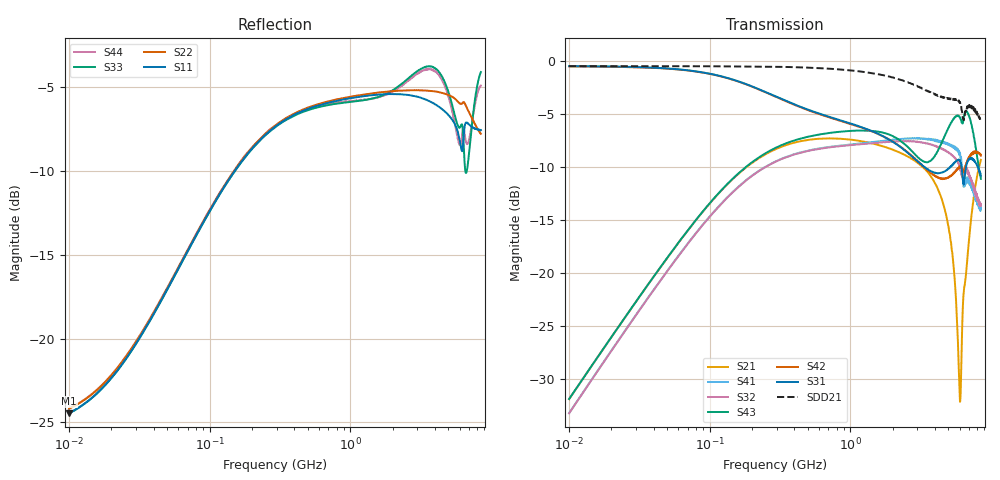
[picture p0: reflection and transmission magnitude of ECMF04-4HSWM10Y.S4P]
!ECMF04-4HSWM10Y
!Typical device
!P1 -OOOOOOO- P3
!P2 -OOOOOOO- P4
!Agilent Technologies,E5071C,MY46109436,A.11.31
!Date: Thu May 02 09:39:07 2019
!Data & Calibration Information:
!Freq	S11:SOLT4(ON)	S12:SOLT4(ON)	S13:SOLT4(ON)	S14:SOLT4(ON)
!	S21:SOLT4(ON)	S22:SOLT4(ON)	S23:SOLT4(ON)	S24:SOLT4(ON)
!	S31:SOLT4(ON)	S32:SOLT4(ON)	S33:SOLT4(ON)	S34:SOLT4(ON)
!	S41:SOLT4(ON)	S42:SOLT4(ON)	S43:SOLT4(ON)	S44:SOLT4(ON)
!PortZ  Port1:50+j0  Port2:50+j0  Port3:50+j0  Port4:50+j0
!Above PortZ is port z conversion or system Z0 setting when saving the data.
!When reading, reference impedance value at option line is always used.
! Lane #1 or Lane #2
# Hz S RI R 50
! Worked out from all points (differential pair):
!   1601 points, 10 MHz to 8.5 GHz, reference 50 ohm
!   strongest paths, dB at 10 MHz, 54.53 MHz, 295.3 MHz, 1.588 GHz, 8.5 GHz:
!     S31: -0.5, -0.7, -3.4, -6.9, -10.8
!     S42: -0.5, -0.8, -3.4, -6.9, -8.9
!     S43: -31.9, -17.9, -8.2, -6.7, -11.1
!     S32: -33.3, -19.2, -9.5, -7.7, -13.7
!     S41: -33.3, -19.1, -9.5, -7.6, -13.9
!     S21: -31.9, -17.9, -8.3, -7.9, -9.3
!   taken as a pair (ports 1,2 in; 3,4 out), SDD21 dB: -0.5, -0.5, -0.5, -1.3, -5.6
!   lowest |S11| = -24.5 dB at 10 MHz (marker M1), VSWR 1.13, Z = 55.7 + j2.72 ohm
!   |S11| at or under -10 dB: start of sweep to 150.4 MHz
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1e7  0.0547 0.0243  0.00222 0.0252  0.9451 -0.0304  -0.00187 -0.0219
     0.00224 0.0252  0.0568 0.0242  -0.0018 -0.0216  0.9426 -0.0306
     0.9449 -0.0306  -0.00183 -0.0216  0.0546 0.0245  0.00201 0.0251
     -0.00182 -0.0216  0.9427 -0.0306  0.00219 0.0252  0.0568 0.0245
6.166333e8  0.499 -0.000887  0.4285 0.0396  0.424 -0.3694  -0.368 0.1153
            0.4279 0.0394  0.5037 0.00474  -0.3712 0.1063  0.4186 -0.3669
            0.4227 -0.3692  -0.3708 0.1062  0.484 0.0916  0.4417 0.0958
            -0.371 0.1117  0.4186 -0.3692  0.4408 0.0943  0.4897 0.0866
1.92501e9  0.3457 -0.4107  0.3434 -0.1759  -0.0322 -0.4257  0.0469 0.4258
           0.3429 -0.1751  0.373 -0.3999  0.0257 0.4176  -0.0265 -0.4255
           -0.0309 -0.4218  0.0237 0.4157  0.5388 -0.0877  0.4276 -0.1308
           0.0414 0.4213  -0.0275 -0.4219  0.4277 -0.1298  0.5326 -0.0958
3.913018e9  -0.2692 -0.4257  0.1283 -0.2392  -0.2869 0.0821  0.4143 -0.0323
            0.13 -0.2397  -0.1982 -0.5102  0.4002 0.00959  -0.2868 0.0573
            -0.2891 0.0736  0.3999 0.0203  0.453 -0.4606  0.3369 -0.0944
            0.4255 -0.0186  -0.2858 0.0505  0.3365 -0.0961  0.4363 -0.459
5.166322e9  -0.4541 -0.0557  -0.00443 -0.1412  -0.052 0.302  0.2273 -0.3176
            -0.00454 -0.1425  -0.4745 -0.2362  0.2541 -0.2505  -0.072 0.2719
            -0.0646 0.3092  0.2672 -0.2457  0.1769 -0.4893  0.4599 -0.2101
            0.2425 -0.3159  -0.0822 0.2736  0.4588 -0.2099  0.1588 -0.475
6.036008e9  -0.3421 0.1825  -0.0245 0.00138  0.1877 0.2663  -0.0502 -0.356
            -0.0245 0.00183  -0.5027 0.0206  0.055 -0.3065  0.1478 0.2743
            0.1903 0.28  0.0655 -0.3104  0.1261 -0.4089  0.3732 -0.3949
            -0.0441 -0.3666  0.1406 0.286  0.3742 -0.3925  0.1286 -0.3568
8.5e9  0.1658 0.385  0.3417 -0.00184  0.2481 -0.0889  -0.1489 0.1192
       0.3411 -0.00954  -0.0989 0.3965  -0.1527 0.1163  0.2613 -0.2008
       0.2706 -0.0974  -0.1685 0.1212  0.0848 -0.6188  0.0275 -0.278
       -0.1548 0.1285  0.2842 -0.2168  0.024 -0.2765  -0.0368 -0.5681
